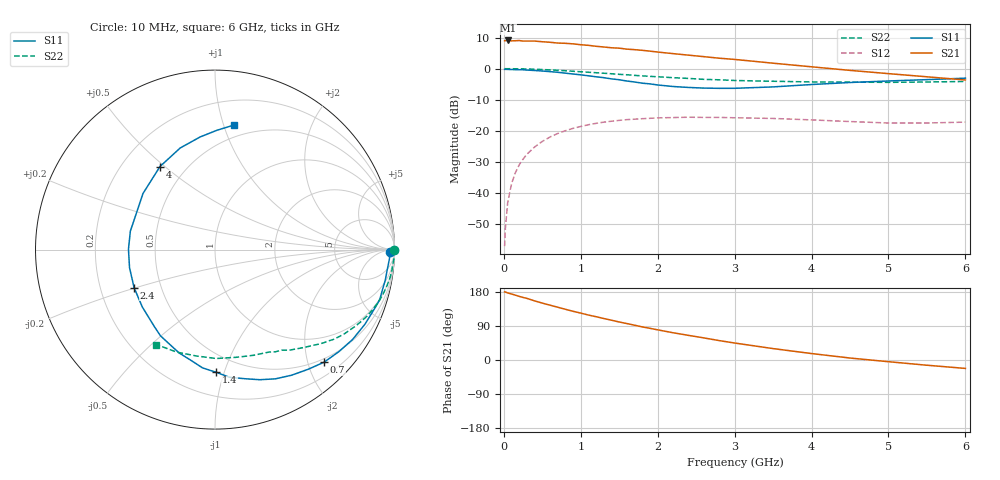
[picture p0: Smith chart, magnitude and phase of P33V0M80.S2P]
! SIEMENS Small Signal Semiconductors
! BFP181
! Si NPN RF Bipolar Junction Transistor in SOT143
! VCE = 3 V  IC = 0.8 mA
! Common Emitter S-Parameters:  March  1996
# GHz  S  MA  R  50
!  f  S11  S21  S12  S22
! GHz  MAG  ANG  MAG  ANG  MAG  ANG  MAG  ANG
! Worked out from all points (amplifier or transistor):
!   36 points, 10 MHz to 6 GHz, reference 50 ohm
!   highest |S21| = 9.1 dB at 50 MHz (marker M1)
!   |S21| within 3 dB of that: start of sweep to 1.72 GHz
!   unconditionally stable (mu >= 1): 3.35 GHz to end of sweep
!   at 250 MHz: K = 0.08, MSG = 19.0 dB, |S12| = -29.1 dB
!   at 1.4 GHz: K = 0.46, MSG = 11.8 dB, |S12| = -16.9 dB
!   at 6 GHz: K = 1.34, MAG = 3.3 dB, |S12| = -17.2 dB
!   S11 on the Smith chart (normalised r, x): 10 MHz: 55, -32; 700 MHz: 0.43, -2.29; 1.4 GHz: 0.37, -0.94; 2.4 GHz: 0.35, -0.20; 4 GHz: 0.36, +0.48; 6 GHz: 0.40, +1.09
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0.01  0.9731 -0.9  2.81 179.7  0.0014 84.2  0.9992 -0.2
0.02  0.9749 -1.4  2.811 179.5  0.0027 90.5  0.9968 -0.6
0.05  0.9728 -3.2  2.837 177.0  0.007 92.4  0.9965 -1.5
0.1  0.9663 -6.6  2.795 174.2  0.0141 83.5  0.9975 -3.2
0.15  0.964 -10.1  2.809 171.1  0.0213 81.8  0.9944 -4.6
0.2  0.9594 -13.6  2.827 167.9  0.0284 80.9  0.9927 -6.3
0.25  0.9593 -16.9  2.771 165.0  0.0352 78.7  0.9902 -7.9
0.4  0.933 -26.5  2.774 156.0  0.055 72.0  0.9774 -12.4
0.7  0.8735 -45.9  2.576 139.3  0.0905 59.3  0.9392 -21.0
0.9  0.8198 -58.6  2.501 128.5  0.1096 51.3  0.9074 -26.2
1.1  0.7667 -71.0  2.367 118.6  0.1255 44.3  0.8743 -30.9
1.4  0.6838 -89.4  2.164 105.0  0.1429 34.6  0.827 -37.3
1.5  0.6627 -96.0  2.133 100.3  0.1473 32.0  0.8098 -39.0
1.8  0.5834 -116.1  1.967 87.3  0.1568 24.6  0.7648 -44.2
2.2  0.516 -141.7  1.742 71.9  0.1635 15.8  0.7157 -50.6
2.4  0.4982 -154.8  1.647 65.0  0.1656 11.8  0.6963 -53.6
3  0.4827 167.7  1.406 44.8  0.1622 2.7  0.6446 -62.4
3.5  0.5085 142.1  1.223 30.1  0.1582 -2.5  0.6265 -70.1
4  0.5552 123.5  1.07 17.0  0.1499 -6.1  0.6113 -79.2
4.5  0.5984 108.9  0.937 5.2  0.1411 -8.2  0.6067 -89.4
5.5  0.6657 88.9  0.739 -13.8  0.1337 -4.2  0.6098 -110.6
6  0.7026 81.2  0.657 -22.2  0.138 -2.2  0.6216 -121.7
